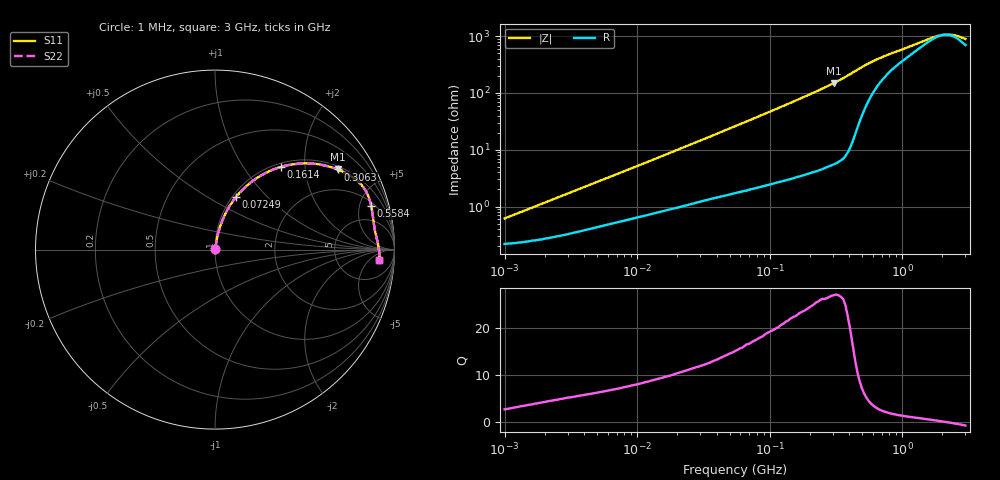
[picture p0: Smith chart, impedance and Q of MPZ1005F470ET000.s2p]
! S-Parameter Data Generated by TDK Corporation
! Copyright(C) 2025 TDK Corporation.
! All Rights Reserved.
! TDK P/N: MPZ1005F470ET000 (Chip Bead)
! Property: |Z|=47ohm at 100MHz
! Size(LxWxT): 1x0.5x0.5mm
! Model Type: s2p (Touchstone File Format Version 1.0)
! Frequency: DC=Yes Start=1MHz Stop=3000MHz 202points Log-sweep
! Model Generated on Feb. 6, 2025
! Terms and conditions regarding TDK Simulation Models:
! 1)This simulation model is being provided solely for informational
!  purposes. Please refer to the specifications of the products in
!  terms of detailed characteristics of such products.
! 2)In no event shall TDK Corporation of any of its subsidiaries be
!  liable for any loss or damage arising, directly or indirectly,
!  from any information contained in this simulation model, including,
!  but not limited to loss or damages arising from any inaccuracies,
!  omissions or errors in connection with such information.
! 3)Any and all copyrights on this simulation model are owned by
!  TDK Corporation.  Duplication or redistribution of this simulation
!  model without prior written permission from TDK Corporation
!  is prohibited.
! 4)This simulation model is subject to any modification or change
!  without any prior notice.
! 5)Neither TDK Corporation nor any of its subsidiaries shall make any
!  warranty, express or implied, including but not limited to the
!  correctness, implied warranties of merchantability and fitness for
!  a particular purpose with respect to this simulation models.
! 6)The use of this simulation model shall be deemed to have consented
!  to the terms and conditions hereof.
! Port Assignments:
!  1 ---@@@--- 2
! Applicable Conditions:
!  Temperature = 25 degC
!  DC Bias Current = 0 A
!  Small Signal Operation
# Hz S MA R 50
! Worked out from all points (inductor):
!   201 points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, 1 MHz to 3 GHz, reference 50 ohm
!   read as one part in series: L = 91.5 nH near 1.222 MHz
!   highest Q = 26.8 at 306.3 MHz (marker M1), where L = 77.6 nH
!   self-resonance near 2.074 GHz
!   S11 on the Smith chart (normalised r, x): 1 MHz: 1.00, +0.01; 72.49 MHz: 1.04, +0.68; 161.4 MHz: 1.07, +1.50; 306.3 MHz: 1.11, +2.99; 558.4 MHz: 2.46, +6.45; 3 GHz: 15, -11
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1000000  0.006176 68.8  0.9978 -0.3  0.9978 -0.3  0.006176 68.8
3900413  0.02154 78.7  0.996 -1.2  0.996 -1.2  0.02154 78.7
1.461624e7  0.07267 79.6  0.9895 -4.1  0.9895 -4.1  0.07267 79.6
3.00453e7  0.1421 77.0  0.978 -8.1  0.978 -8.1  0.1421 77.0
5.477226e7  0.2463 72.0  0.9529 -14.2  0.9529 -14.2  0.2463 72.0
7.248696e7  0.3157 68.2  0.9303 -18.4  0.9303 -18.4  0.3157 68.2
1.081723e8  0.4403 61.0  0.8757 -26.1  0.8757 -26.1  0.4403 61.0
1.614254e8  0.5884 51.5  0.783 -36.0  0.783 -36.0  0.5884 51.5
2.136344e8  0.6947 43.7  0.6919 -44.0  0.6919 -44.0  0.6947 43.7
2.507343e8  0.7521 39.1  0.6308 -48.7  0.6308 -48.7  0.7521 39.1
3.062963e8  0.8172 33.1  0.5468 -54.8  0.5468 -54.8  0.8172 33.1
3.594878e8  0.8627 28.3  0.4737 -59.5  0.4737 -59.5  0.8627 28.3
4.219165e8  0.8954 23.2  0.3945 -63.3  0.3945 -63.3  0.8954 23.2
4.75755e8  0.9041 19.6  0.3369 -63.9  0.3369 -63.9  0.9041 19.6
5.583748e8  0.9035 15.5  0.2734 -61.8  0.2734 -61.8  0.9035 15.5
8.005644e8  0.8964 9.4  0.1866 -51.7  0.1866 -51.7  0.8964 9.4
1.645649e9  0.9082 2.2  0.09888 -20.7  0.09888 -20.7  0.9082 2.2
1.931433e9  0.9121 0.7  0.08864 -7.1  0.08864 -7.1  0.9121 0.7
2.177892e9  0.9146 -0.5  0.0858 5.2  0.0858 5.2  0.9146 -0.5
2.359433e9  0.9159 -1.3  0.08675 13.6  0.08675 13.6  0.9159 -1.3
2.660507e9  0.9171 -2.5  0.0926 25.3  0.0926 25.3  0.9171 -2.5
3e9  0.9171 -3.7  0.1034 34.9  0.1034 34.9  0.9171 -3.7
